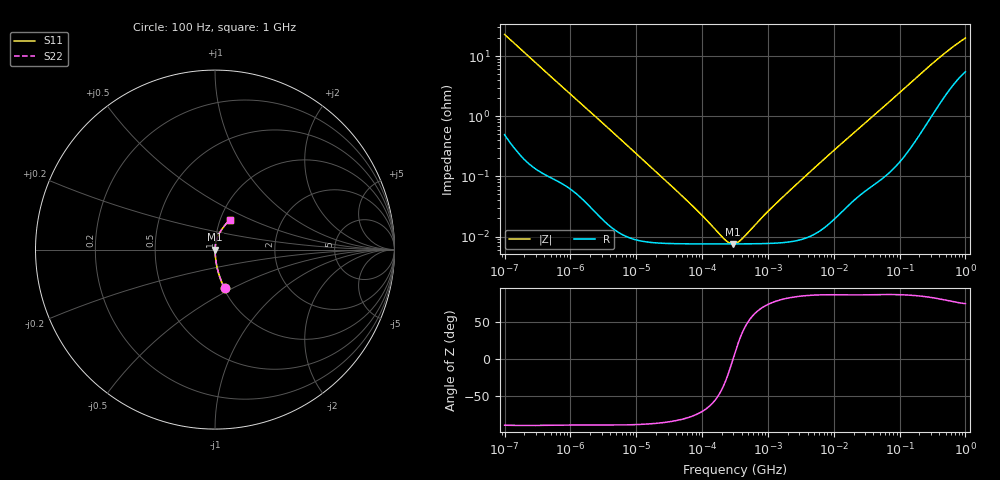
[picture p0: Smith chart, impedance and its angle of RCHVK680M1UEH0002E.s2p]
! RCHVK680M1UEH0002E  S-PARAMETER MODEL  (AEC-Q200 qualified)
! Model Generated by ELNA Corporation (http://www.ty-top.com)
! Version 1.0
! ELNA Control No. 240315
! Copyright (c) 2024 ELNA CO.,LTD. All Rights Reserved.
! Products Name : CONDUCTIVE POLYMER HYBRID ALUMINUM ELECTROLYTIC CAPACITORS
! Characteristics :
!  Capacitance  :  68uF  ,  Rated voltage  :  50V
!  Operating Temp. Range  :  -55 to +125 degC  ,  Endurance  :  4000hr at 125 degC
!  Dimension D  :  8mm  ,  Dimension L  :  10mm
! Frequency Range : 100Hz - 1GHz
! External Node Assignments :
!  1  o---| |---o  2
# MHz S RI R 50
!Freq[MHz].  S11 Real  S11 Imag  S21 Real  S21 Imag  S12 Real  S12 Imag  S22 Real  S22 Imag
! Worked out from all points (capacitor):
!   401 points, 100 Hz to 1 GHz, reference 50 ohm
!   read as one part in series: C = 69.6 uF near 108 Hz
!   lowest |Z| = 7.53 mohm at 291.7 kHz (marker M1)
!   series resonance near 295.5 kHz, so ESL is about 4.2 nH
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0.0001  0.0539 -0.2153  0.9461 0.2153  0.9461 0.2153  0.0539 -0.2153
0.000113  0.043 -0.1931  0.957 0.1931  0.957 0.1931  0.043 -0.1931
0.000183  0.0174 -0.1226  0.9826 0.1226  0.9826 0.1226  0.0174 -0.1226
0.000309  0.00674 -0.0736  0.9933 0.0736  0.9933 0.0736  0.00674 -0.0736
0.000613  0.00226 -0.0375  0.9977 0.0375  0.9977 0.0375  0.00226 -0.0375
0.001488  0.000675 -0.0158  0.9993 0.0158  0.9993 0.0158  0.000675 -0.0158
0.022131  7.89e-05 -0.00107  0.9999 0.00107  0.9999 0.00107  7.89e-05 -0.00107
0.080353  7.54e-05 -0.000275  0.9999 0.000275  0.9999 0.000275  7.54e-05 -0.000275
0.187284  7.53e-05 -7.62e-05  0.9999 7.62e-05  0.9999 7.62e-05  7.53e-05 -7.62e-05
0.211349  7.53e-05 -5.51e-05  0.9999 5.51e-05  0.9999 5.51e-05  7.53e-05 -5.51e-05
0.291743  7.53e-05 -2.01e-06  0.9999 2.01e-06  0.9999 2.01e-06  7.53e-05 -2.01e-06
0.316228  7.53e-05 1.1e-05  0.9999 -1.1e-05  0.9999 -1.1e-05  7.53e-05 1.1e-05
0.419276  7.54e-05 5.78e-05  0.9999 -5.78e-05  0.9999 -5.78e-05  7.54e-05 5.78e-05
0.473151  7.55e-05 7.9e-05  0.9999 -7.9e-05  0.9999 -7.9e-05  7.55e-05 7.9e-05
0.767361  7.6e-05 0.000179  0.9999 -0.000179  0.9999 -0.000179  7.6e-05 0.000179
1.148154  7.71e-05 0.000293  0.9999 -0.000293  0.9999 -0.000293  7.71e-05 0.000293
4.704354  0.000106 0.00128  0.9999 -0.00128  0.9999 -0.00128  0.000106 0.00128
69.9842  0.00145 0.0173  0.9986 -0.0173  0.9986 -0.0173  0.00145 0.0173
176.8072  0.00576 0.0426  0.9942 -0.0426  0.9942 -0.0426  0.00576 0.0426
380.1894  0.0216 0.0853  0.9784 -0.0853  0.9784 -0.0853  0.0216 0.0853
668.3439  0.0509 0.1305  0.9491 -0.1305  0.9491 -0.1305  0.0509 0.1305
1000  0.0824 0.167  0.9176 -0.167  0.9176 -0.167  0.0824 0.167
